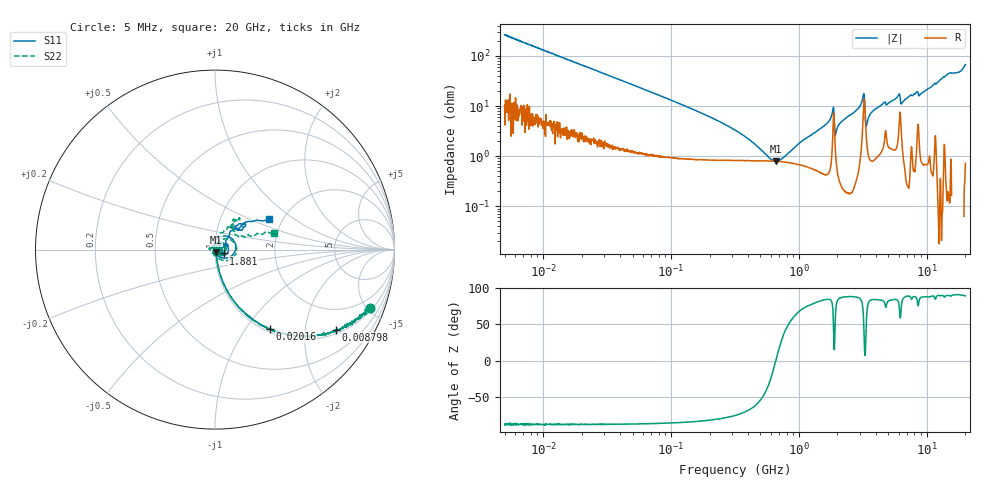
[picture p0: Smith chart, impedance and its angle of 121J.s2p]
!Keysight Technologies,P5008B,MY61100088,A.16.20.02
!Date: Wednesday, November 08, 2023 15:29:24
!Correction: S11(C  2-Port  )
!S21(C  2-Port  )
!S12(C  2-Port  )
!S22(C  2-Port  )
!S2P File: Measurements: S11, S21, S12, S22:Log Frequency Sweep
# Hz S  dB  R 50
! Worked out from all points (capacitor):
!   1601 points, 5 MHz to 20 GHz, reference 50 ohm
!   read as one part in series: C = 121 pF near 5.212 MHz
!   lowest |Z| = 795 mohm at 660.2 MHz (marker M1)
!   series resonance near 659.4 MHz, so ESL is about 480 pH
!   S11 on the Smith chart (normalised r, x): 5 MHz: 1.20, -5.27; 8.798 MHz: 1.13, -2.93; 20.16 MHz: 1.05, -1.30; 1.881 GHz: 1.10, -0.05; 20 GHz: 1.71, +0.65
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5000000  -0.69 -20.5  -9.11 67.3  -9.11 67.3  -0.69 -20.5
8797522  -1.84 -33.5  -5.16 53.8  -5.16 53.9  -1.84 -33.5
1.995555e7  -5.26 -55.1  -1.72 33.0  -1.72 33.0  -5.26 -55.1
2.016352e7  -5.40 -55.4  -1.69 32.4  -1.69 32.4  -5.41 -55.4
7.964482e7  -15.70 -77.3  -0.20 9.2  -0.20 9.2  -15.76 -77.5
3.162278e8  -27.85 -76.5  -0.08 1.5  -0.08 1.5  -28.85 -76.7
6.602111e8  -35.18 -67.1  -0.08 -0.7  -0.08 -0.7  -40.06 -52.3
9.392266e8  -39.76 -63.2  -0.08 -1.8  -0.08 -1.8  -47.64 13.7
1.2621e9  -46.93 -68.2  -0.09 -2.9  -0.09 -2.9  -43.62 81.5
1.429304e9  -61.87 154.7  -0.09 -3.5  -0.09 -3.5  -39.78 85.8
1.881234e9  -25.60 -24.4  -0.58 -3.2  -0.58 -3.2  -25.74 -20.7
2.022837e9  -46.70 -156.6  -0.11 -4.6  -0.11 -4.6  -45.59 143.3
3.175579e9  -20.40 52.7  -0.62 -11.7  -0.62 -11.7  -20.68 40.2
3.633761e9  -48.77 124.4  -0.12 -8.2  -0.13 -8.2  -42.17 -36.8
4.588432e9  -32.33 61.8  -0.14 -11.8  -0.14 -11.8  -29.39 32.3
5.037181e9  -35.94 52.4  -0.12 -12.4  -0.13 -12.4  -30.82 19.5
6.102182e9  -23.35 22.6  -0.54 -16.8  -0.54 -16.8  -25.49 14.9
8.031625e9  -50.83 34.3  -0.11 -20.1  -0.11 -20.1  -45.26 148.6
8.771529e9  -30.32 -68.2  -0.14 -20.7  -0.14 -20.7  -30.93 -101.0
1.014171e10  -30.90 -22.3  -0.03 -25.8  -0.04 -25.8  -42.26 146.0
1.369891e10  -15.23 40.3  -0.24 -36.9  -0.24 -36.8  -16.40 52.6
2e10  -9.19 29.0  -0.68 -66.8  -0.69 -66.8  -9.35 15.3
